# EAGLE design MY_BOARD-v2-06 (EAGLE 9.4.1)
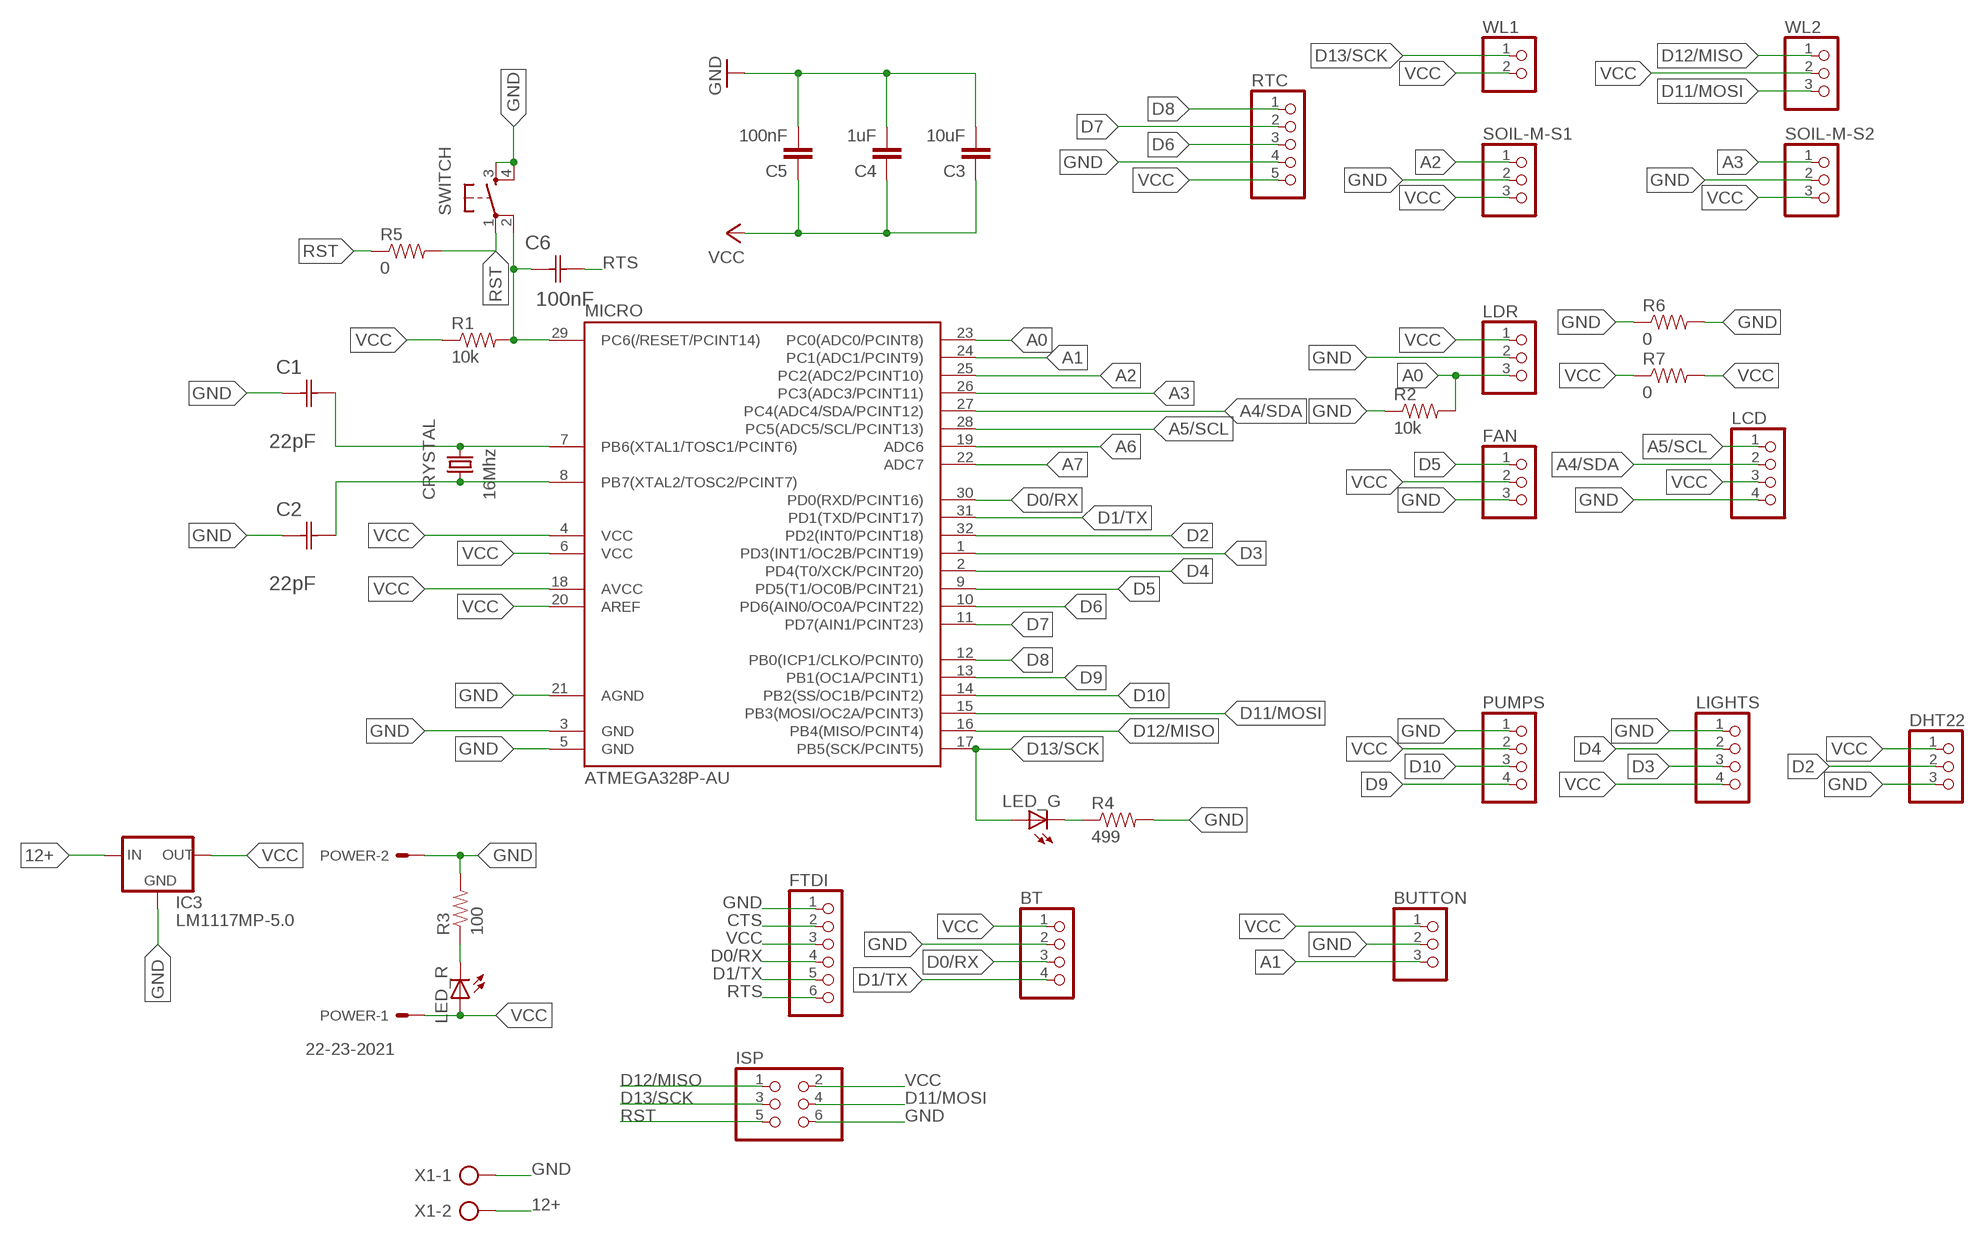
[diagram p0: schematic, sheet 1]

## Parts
BT  PINHD-1X4/90  [1X04/90]
BUTTON  PINHD-1X3/90  [1X03/90]
C1  22pF  0612ZC225MAT2A  [CAPC3216X178N]
C2  22pF  0612ZC225MAT2A  [CAPC3216X178N]
C3  10uF  CAP1206  [1206]
C4  1uF  CAP1206  [1206]
C5  100nF  CAP1206  [1206]
C6  100nF  0612ZC225MAT2A  [CAPC3216X178N]
CRYSTAL  16Mhz  CSM-7X-DU  [CSM-7X-DU]
DHT22  PINHD-1X3/90  [1X03/90]
FAN  PINHD-1X3/90  [1X03/90]
FTDI  PINHD-1X6  [1X06]
IC3  LM1117MP-5.0  [SOT223]
ISP  PINHD-2X3-SMD  [2X03SMD]
LCD  PINHD-1X4/90  [1X04/90]
LDR  PINHD-1X3/90  [1X03/90]
LED_G  LED1206  [1206]
LED_R  LED1206  [1206]
LIGHTS  PINHD-1X4/90  [1X04/90]
MICRO  ATMEGA328P-AU  ATMEGA48/88/168-AU  [TQFP32-08]
POWER  22-23-2021  [22-23-2021]
PUMPS  PINHD-1X4/90  [1X04/90]
R1  10k  RESISTOR1206  [1206]
R2  10k  RESISTOR1206  [1206]
R3  100  RESISTOR1206  [1206]
R4  499  RESISTOR1206  [1206]
R5  0  RESISTOR1206  [1206]
R6  0  RESISTOR1206  [1206]
R7  0  RESISTOR1206  [1206]
RTC  PINHD-1X5/90  [1X05/90]
SOIL-M-S1  PINHD-1X3/90  [1X03/90]
SOIL-M-S2  PINHD-1X3/90  [1X03/90]
SWITCH  6MM_SWITCH6MM_SWITCH  [6MM_SWITCH]
WL1  PINHD-1X2/90  [1X02/90]
WL2  PINHD-1X3/90  [1X03/90]
X1  AK500/2  [AK500/2]

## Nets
12+: IC3.3(IN) X1.2
A0: LDR.3 MICRO.23(PC0(ADC0/PCINT8)) R2.2
A1: BUTTON.3 MICRO.24(PC1(ADC1/PCINT9))
A2: MICRO.25(PC2(ADC2/PCINT10)) SOIL-M-S1.1
A3: MICRO.26(PC3(ADC3/PCINT11)) SOIL-M-S2.1
A4/SDA: LCD.2 MICRO.27(PC4(ADC4/SDA/PCINT12))
A5/SCL: LCD.1 MICRO.28(PC5(ADC5/SCL/PCINT13))
A6: MICRO.19(ADC6)
A7: MICRO.22(ADC7)
CTS: FTDI.2
D0/RX: BT.3 FTDI.4 MICRO.30(PD0(RXD/PCINT16))
D1/TX: BT.4 FTDI.5 MICRO.31(PD1(TXD/PCINT17))
D2: DHT22.2 MICRO.32(PD2(INT0/PCINT18))
D3: LIGHTS.3 MICRO.1(PD3(INT1/OC2B/PCINT19))
D4: LIGHTS.2 MICRO.2(PD4(T0/XCK/PCINT20))
D5: FAN.1 MICRO.9(PD5(T1/OC0B/PCINT21))
D6: MICRO.10(PD6(AIN0/OC0A/PCINT22)) RTC.3
D7: MICRO.11(PD7(AIN1/PCINT23)) RTC.2
D8: MICRO.12(PB0(ICP1/CLKO/PCINT0)) RTC.1
D9: MICRO.13(PB1(OC1A/PCINT1)) PUMPS.4
D10: MICRO.14(PB2(SS/OC1B/PCINT2)) PUMPS.3
D11/MOSI: ISP.4 MICRO.15(PB3(MOSI/OC2A/PCINT3)) WL2.3
D12/MISO: ISP.1 MICRO.16(PB4(MISO/PCINT4)) WL2.1
D13/SCK: ISP.3 LED_G.1(A) MICRO.17(PB5(SCK/PCINT5)) WL1.1
GND: BT.2 BUTTON.2 C1.1(C1) C2.1(C1) C3.2 C4.2 C5.2 DHT22.3 FAN.3 FTDI.1 IC3.1(GND) ISP.6 LCD.4 LDR.2 LIGHTS.1 MICRO.3(GND) MICRO.5(GND) MICRO.21(AGND) POWER.2 PUMPS.1 R2.1 R3.2 R4.2 R6.1 R6.2 RTC.4 SOIL-M-S1.2 SOIL-M-S2.2 SWITCH.3(S) SWITCH.4(S1) X1.1
LED: LED_R.2(C) R3.1
LED1: LED_G.2(C) R4.1
RST: C6.1(C1) ISP.5 MICRO.29(PC6(/RESET/PCINT14)) R1.2 R5.1 R5.2 SWITCH.1(P) SWITCH.2(P1)
RTS: C6.2(C2) FTDI.6
VCC: BT.1 BUTTON.1 C3.1 C4.1 C5.1 DHT22.1 FAN.2 FTDI.3 IC3.2(OUT) IC3.4(OUT) ISP.2 LCD.3 LDR.1 LED_R.1(A) LIGHTS.4 MICRO.4(VCC) MICRO.6(VCC) MICRO.18(AVCC) MICRO.20(AREF) POWER.1 PUMPS.2 R1.1 R7.1 R7.2 RTC.5 SOIL-M-S1.3 SOIL-M-S2.3 WL1.2 WL2.2
XTAL1: C1.2(C2) CRYSTAL.2 MICRO.7(PB6(XTAL1/TOSC1/PCINT6))
XTAL2: C2.2(C2) CRYSTAL.1 MICRO.8(PB7(XTAL2/TOSC2/PCINT7))

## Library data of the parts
BT LCD LIGHTS PUMPS = pinhead:PINHD-1X4: PIN HEADER
BUTTON DHT22 FAN LDR SOIL-M-S1 SOIL-M-S2 WL2 = pinhead:PINHD-1X3: PIN HEADER
C1 C2 C6 = AVX_By_element14_Batch_1:0612ZC225MAT2A: Capacitor 1206; MPN: 0612ZC225MAT2A; OC_FARNELL: -; OC_NEWARK: 12N3209; SUPPLIER: AVX; TOLERANCE: ±20%; VALUE: 2.2µF; VOLTAGERATING: 10V
C3-C5 = 01_SparkFun:CAP: Capacitor
CRYSTAL = 01_FAB_Hello:CSM-7X-DU: SMD CRYSTAL; OC_FARNELL: unknown; OC_NEWARK: unknown
FTDI = pinhead:PINHD-1X6: PIN HEADER
IC3 = lm1117:LM1117?-*: 800mA Low-Dropout Linear Regulator Source: http://ww1.microchip.com/downloads/en/DeviceDoc/39760d.pdf; MF: Texas Instruments; MPN: LM1117MP-5.0; OC_FARNELL: 9778209; OC_NEWARK: 28X3417; SPICEPREFIX: J
ISP = fab:PINHD-2X3-SMD: PIN HEADER
LED_G LED_R = 01_FAB_Hello:LED
MICRO = atmega8:ATMEGA48/88/168
POWER = con-molex:22-23-2021: .100" (2.54mm) Center Header - 2 Pin; MF: MOLEX; MPN: 22-23-2021; OC_FARNELL: 1462926; OC_NEWARK: 25C3832
R1-R7 = 01_SparkFun:RESISTOR: Resistor
RTC = pinhead:PINHD-1X5: PIN HEADER
SWITCH = 01_FAB_Hello:6MM_SWITCH: OMRON SWITCH
WL1 = pinhead:PINHD-1X2: PIN HEADER
X1 = con-ptr500:AK500/2: CONNECTOR; OC_FARNELL: unknown; OC_NEWARK: unknown

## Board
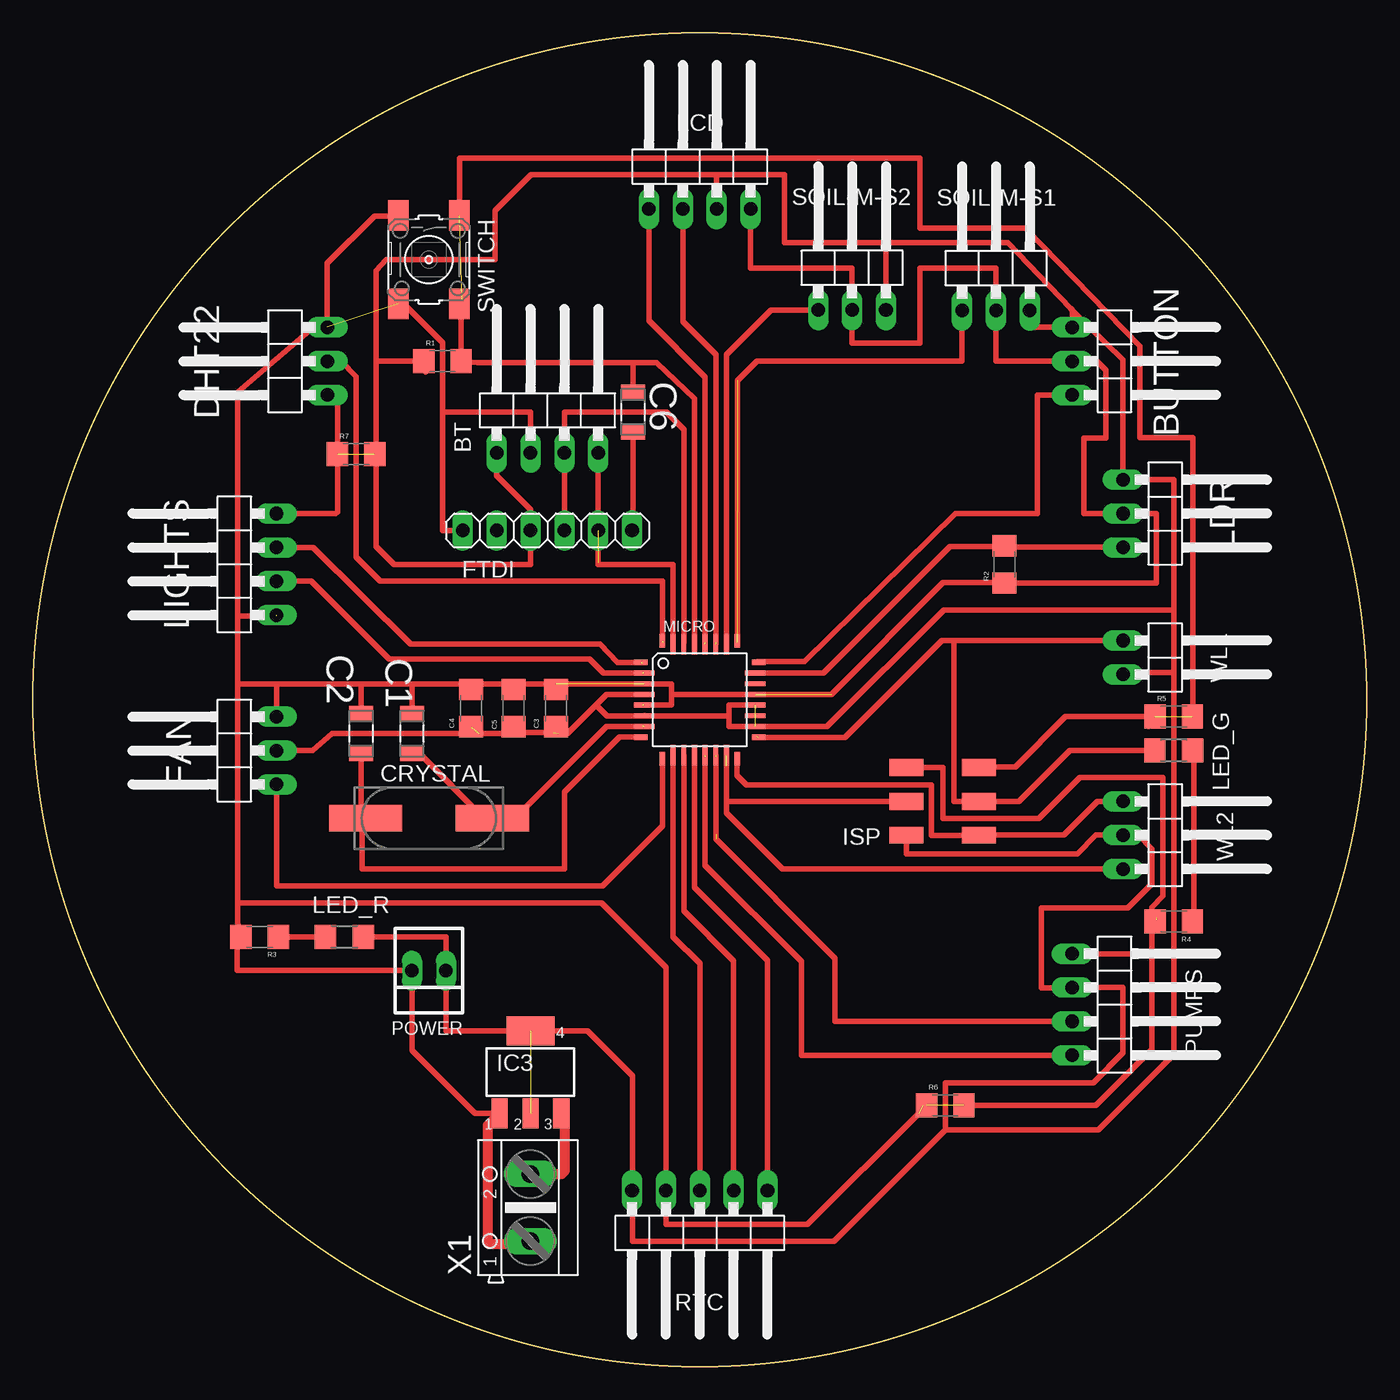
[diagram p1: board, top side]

Size 100 x 100 mm. Coordinates in mm from the lower left corner, seen from the top.
Outline: circle at 50,50 radius 50
Copper layers (1*16): Top 0.035mm / dielectric 1.5mm / Bottom 0.035mm
Design rules "default *": minimum track width 16mil, minimum drill 0.35mm, track to track 16mil, track to pad 16mil, pad to pad 16mil, via to via 16mil, smd to smd 6mil, copper to edge 40mil, drill to drill 6mil, minimum pad ring 10mil, minimum via ring 8mil, stop-mask expansion 4mil, vias tented up to drill 0mil, thermal gap 10mil

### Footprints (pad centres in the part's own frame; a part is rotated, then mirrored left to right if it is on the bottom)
1X04/90 = drill 1.016 long: 1 -3.81,-3.81; 2 -1.27,-3.81; 3 1.27,-3.81; 4 3.81,-3.81
1X03/90 = drill 1.016 long: 1 -2.54,-3.81; 2 0,-3.81; 3 2.54,-3.81
CAPC3216X178N = smd 1.118 x 1.803: 1 -1.499,0; 2 1.499,0
1206 = smd 1.6 x 1.8: 1 -1.4,0; 2 1.4,0
CSM-7X-DU = smd 5.5 x 2: 1 -4.75,0; 2 4.75,0
1X06 = drill 1.016 long: 1 -6.35,0; 2 -3.81,0; 3 -1.27,0; 4 1.27,0; 5 3.81,0; 6 6.35,0
SOT223 = smd 1.219 x 2.235: 1 -2.311,-3.099; 2 0,-3.099; 3 2.311,-3.099 | smd 3.6 x 2.2: 4 0,3.099
2X03SMD = smd 2.54 x 1.27: 1 -2.54,2.54; 2 2.92,2.54; 3 -2.54,0; 4 2.92,0; 5 -2.54,-2.54; 6 2.92,-2.54
1206' = smd 1.6 x 1.803: 1 -1.422,0; 2 1.422,0
TQFP32-08 = smd 1.016 x 0.406: 1 -4.42,2.8; 8 -4.42,-2.8; 17 4.42,-2.8; 24 4.42,2.8 | smd 1.524 x 0.356: 2 -4.166,2; 3 -4.166,1.2; 4 -4.166,0.4; 5 -4.166,-0.4; 6 -4.166,-1.2; 7 -4.166,-2; 18 4.166,-2; 19 4.166,-1.2; 20 4.166,-0.4; 21 4.166,0.4; 22 4.166,1.2; 23 4.166,2 | smd 0.406 x 1.016: 9 -2.8,-4.42; 16 2.8,-4.42; 25 2.8,4.42; 32 -2.8,4.42 | smd 0.356 x 1.524: 10 -2,-4.166; 11 -1.2,-4.166; 12 -0.4,-4.166; 13 0.4,-4.166; 14 1.2,-4.166; 15 2,-4.166; 26 2,4.166; 27 1.2,4.166; 28 0.4,4.166; 29 -0.4,4.166; 30 -1.2,4.166; 31 -2,4.166
22-23-2021 = drill 1 long: 1 -1.27,0; 2 1.27,0
1X05/90 = drill 1.016 long: 1 -5.08,-3.81; 2 -2.54,-3.81; 3 0,-3.81; 4 2.54,-3.81; 5 5.08,-3.81
6MM_SWITCH = smd 2.286 x 1.524: 1 -3.302,2.286; 2 3.302,2.286; 3 -3.302,-2.286; 4 3.302,-2.286
1X02/90 = drill 1.016 long: 1 -1.27,-3.81; 2 1.27,-3.81
AK500/2 = drill 1.321 long: 1 -2.515,0; 2 2.515,0

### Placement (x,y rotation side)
BT  38.57,72.35 0 top
BUTTON  81.75,75.4 270 top
C1  28.41,47.46 270 top
C2  24.6,47.46 270 top
C3  39.2,49.37 90 top
C4  32.86,49.37 90 top
C5  36.03,49.37 90 top
C6  45,71.59 270 top
CRYSTAL  29.68,41.11 0 top
DHT22  18.25,75.4 90 top
FAN  14.44,46.19 90 top
FTDI  38.57,62.7 0 top
IC3  37.3,22.06 0 top
ISP  68.41,42.38 180 top
LCD  50,90.64 0 top
LDR  85.56,63.97 270 top
LED_G  [1206']  85.56,46.19 0 top
LED_R  [1206']  23.33,32.22 180 top
LIGHTS  14.44,60.16 90 top
MICRO  50,50 0 top
POWER  29.68,29.68 180 top
PUMPS  81.75,27.14 270 top
R1  30.7,75.4 0 top
R2  72.86,60.16 90 top
R3  16.98,32.22 180 top
R4  85.56,33.36 180 top
R5  85.56,48.73 0 top
R6  68.41,19.57 0 top
R7  24.22,68.41 0 top
RTC  50,9.36 180 top
SOIL-M-S1  72.22,83.02 0 top
SOIL-M-S2  61.43,83.05 0 top
SWITCH  29.68,83.02 270 top
WL1  85.56,53.17 270 top
WL2  85.56,39.84 270 top
X1  37.3,11.9 90 top

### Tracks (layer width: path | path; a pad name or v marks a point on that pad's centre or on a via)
12+
  Top 0.406: 39.66,14.41 39.84,14.59
  Top 0.762: IC3.3 39.84,18.73 39.84,14.59 | X1.2 39.66,14.41
A0
  Top 0.406: MICRO.23 59.27,52 68.75,61.48 72.88,61.48 R2.2 | 73.07,61.2 R2.2 | LDR.3 81.72,61.46 73.01,61.46 R2.2
A1
  Top 0.406: BUTTON.3 75.32,72.86 75.32,63.97 69.18,63.97 57.86,52.85 54.34,52.85 54.29,52.8
A2  (1 unrouted)
  Top 0.406: 52.82,54.42 52.82,73.93 54.29,75.4 69.69,75.4 SOIL-M-S1.1
A3
  Top 0.406: SOIL-M-S2.1 55.34,79.23 52,75.89 52,54.29
A4/SDA  (1 unrouted)
  Top 0.406: MICRO.27 51.2,75.91 48.73,78.38 LCD.2
A5/SCL  (1 unrouted)
  Top 0.406: MICRO.28 50.4,74.22 46.19,78.43 LCD.1
D0/RX
  Top 0.406: 48.8,54.29 48.8,70.27 47.5,71.59 39.84,71.59 39.84,68.92 BT.3 | BT.3 39.82,67.93 | FTDI.4 BT.3
D1/TX  (1 unrouted)
  Top 0.406: 48,54.29 48,60.16 42.38,60.16 FTDI.5 | BT.4 42.38,60.29
D2  (1 unrouted)
  Top 0.406: DHT22.2 23.08,75.4 24.22,74.26 24.22,60.69 26.02,58.89 47.2,58.89 MICRO.32
D3  (1 unrouted)
  Top 0.406: LIGHTS.3 21,61.43 28.32,54.19 42.51,54.19 43.82,52.8 MICRO.1
D4  (1 unrouted)
  Top 0.406: LIGHTS.2 20.84,58.89 26.68,53.05 41.72,53.05 42.77,52 MICRO.2
D5
  Top 0.406: FAN.1 18.25,36.03 42.72,36.03 47.2,40.51 47.2,45.71
D6
  Top 0.406: RTC.3 50,30.21 48,32.21 MICRO.10
D7
  Top 0.406: MICRO.11 48.8,34.15 52.54,30.41 RTC.2
D8
  Top 0.406: 49.61,45.82 MICRO.12 49.6,35.92 55.08,30.44 RTC.1
D9  (1 unrouted)
  Top 0.406: PUMPS.4 57.62,23.33 57.62,30.37 50.4,37.59 MICRO.13
D10  (2 unrouted)
  Top 0.406: MICRO.14 51.2,39.91 | PUMPS.3 60.16,25.87 60.16,30.59 51.21,39.54 51.21,39.91
D11/MOSI  (1 unrouted)
  Top 0.406: ISP.4 52,42.38 | 52,45.03 52,42.38 | 52,42.38 52,41.52 56.22,37.3 WL2.3
D12/MISO
  Top 0.406: MICRO.16 52.8,44.34 53.51,43.62 67.37,43.62 67.37,39.83 69.8,39.83 ISP.1 77.31,39.84 79.84,42.38 WL2.1
D13/SCK  (1 unrouted)
  Top 0.406: 69.08,54.45 69.08,42.38 ISP.3 73.95,42.38 77.76,46.19 LED_G.1 | 54.42,47.19 60.9,47.19 68.16,54.45 69.08,54.45 | 69.08,54.45 WL1.1
GND  (9 unrouted)
  Top 0.406: 24.6,51.2 18.38,51.2 | 18.38,51.2 15.33,51.2 | C2.1 24.6,51.2 | C1.1 28.41,51.2 | 39.2,51.2 36.66,51.2 | 36.66,51.2 33.36,51.2 | 15.33,34.76 15.33,51.2 | 30.7,71.59 30.7,62.7 FTDI.1 | 30.7,71.59 30.7,76.8 27.8,79.72 SWITCH.4 | SWITCH.3 27.95,86.3 25.61,86.3 22.06,82.75 DHT22.3 21.02,77.94 15.33,73.09 15.33,56.3 | 83.91,30.95 83.91,23.76 79.72,19.57 R6.2 | 18.25,56.3 15.33,56.3 | 15.33,34.76 42.63,34.76 47.46,29.93 RTC.4 47.46,10.63 58.1,10.63 66.41,18.94 | ISP.6 68.24,44.92 68.24,41.11 75.45,41.11 78.52,44.18 84.74,44.18 84.74,35.27 83.91,34.43 83.91,33.24 | R6.1 66.76,19.57 | 15.33,34.76 15.33,33.24 R3.2 15.27,31.91 15.27,29.68 POWER.2 28.41,23.71 33.16,18.96 IC3.1 | PUMPS.1 83.91,30.95 | 84.29,33.49 R4.2 | FAN.3 18.25,51.07 18.38,51.2 | 15.33,56.3 15.33,51.2 | 83.91,30.95 83.91,33.24 | 83.91,33.24 84.29,33.62 | C4.2 33.36,50.64 33.36,51.2 | 33.36,51.2 33.36,51.23 | C5.2 36.66,51.2 | C3.2 39.2,51.2 | 47.88,50.4 59.87,50.4 68.26,58.78 72.84,58.78 R2.1 72.87,58.74 84.27,58.74 84.27,63.97 LDR.2 78.8,63.97 78.8,69.63 80.48,69.63 80.48,74.75 79.78,75.4 BUTTON.2 72.22,75.4 SOIL-M-S1.2 72.22,82.38 66.51,82.38 66.51,76.77 61.43,76.77 SOIL-M-S2.2 61.43,82.38 53.81,82.38 LCD.4 | 45.71,49.6 47.84,49.6 47.88,49.64 47.88,50.4 | 39.2,51.2 47.88,51.2 47.88,50.4 | 30.7,71.59 37.3,71.59 BT.2 37.28,68.56 | 24.6,51.2 28.41,51.2 | 28.41,51.2 33.36,51.2 | 37.1,9.18 X1.1
  Top 0.762: IC3.1 34.1,18.07 34.1,9.18 37.1,9.18
LED
  Top 0.406: R3.1 LED_R.2
LED1
  Top 0.406: 86.98,45.43 LED_G.2 86.83,46.17 87.09,45.91 87.09,33.49 R4.1 86.98,33.39
RST  (2 unrouted)
  Top 0.406: 32.15,79.94 SWITCH.2 32.1,79.59 R1.2 33.33,75.3 45.02,75.3 | 45.02,75.3 46.75,75.3 49.6,72.6 49.6,54.29 | ISP.5 70.12,44.97 73.67,44.97 77.43,48.73 R5.1 83.66,47.98 | SWITCH.1 31.97,90.64 66.51,90.64 66.51,85.37 74.45,85.37 83.02,76.54 83.02,69.69 87.01,69.69 87.01,48.74 R5.2 | C6.1 45,75.27 45.02,75.3
RTS
  Top 0.406: 44.95,70.04 C6.2 45,62.78 FTDI.6
VCC  (5 unrouted)
  Top 0.406: 54.18,49.59 MICRO.20 52.21,49.6 52.21,48.8 | 45.85,48.81 MICRO.6 | 85.56,56.73 68.33,56.73 59.53,48 52.21,48 52.21,48.8 | 29.43,74.59 R1.1 25.72,75.4 | MICRO.4 45.83,50.38 42.99,50.38 42.23,49.62 | MICRO.6 52.21,48.8 | 44.95,15.73 RTC.5 44.95,15.69 | 85.56,52.03 85.56,23.38 79.9,17.72 68.41,17.72 | 85.56,56.73 85.56,52.03 | 68.41,17.72 68.41,21.27 79.52,21.27 81.75,23.51 81.75,28.41 PUMPS.2 77.95,28.39 75.63,28.39 75.63,34.38 82.12,34.38 83.92,36.19 83.92,38.81 82.89,39.84 WL2.2 79.72,39.84 78.32,38.44 65.49,38.44 65.5,38.44 ISP.2 | 44.95,15.69 44.95,9.36 60.06,9.36 68.41,17.72 | BUTTON.1 79.22,77.94 81.75,75.52 LDR.1 85.56,66.51 85.56,56.73 | 79.18,77.94 77.81,79.37 | 77.81,79.37 73.11,84.29 63.97,84.29 | FTDI.3 37.27,61.4 | POWER.1 30.95,25.16 IC3.4 | BUTTON.1 74.77,77.94 SOIL-M-S1.3 | WL1.2 81.88,52.03 85.56,52.03 | 25.72,75.4 25.72,82.2 26.46,83.02 34.63,83.02 34.63,86.7 37.33,89.4 51.3,89.4 | LIGHTS.4 22.7,63.97 22.82,64.1 R7.1 | 22.7,72.86 22.82,72.86 R7.1 | 22.7,72.86 DHT22.1 | FAN.2 20.95,46.19 22.42,47.46 33.44,47.46 | 33.44,47.46 33.52,47.49 | POWER.1 30.95,32.22 LED_R.1 | 44.95,15.69 44.95,21.78 41.57,25.16 IC3.4 | 42.23,49.62 40.09,47.48 39.69,47.48 C3.1 39.37,47.8 39.37,47.48 | 42.23,49.62 43.05,48.8 MICRO.6 | IC3.4 36.59,25.87 | 30.95,25.87 POWER.1 | 22.82,72.74 22.7,72.86 | BUTTON.1 77.94,79.24 77.81,79.37 | BT.1 34.76,66.81 37.3,64.27 FTDI.3 | R7.1 | 25.87,68.67 25.72,68.51 | 25.72,68.51 R7.2 | SOIL-M-S2.3 63.97,84.29 | 51.3,89.4 51.27,89.37 LCD.3 | FTDI.3 37.3,60.16 27.06,60.16 25.72,61.51 25.72,68.51 | 25.72,75.4 25.72,68.51 | 33.44,47.46 35.78,47.46 C5.1 36.21,47.53 39.03,47.53
  Top 0.406: 51.3,89.4 56.35,89.4 56.35,84.29 63.97,84.29
XTAL1  (1 unrouted)
  Top 0.406: MICRO.7 43.02,48 36.18,41.16 35.32,41.16 CRYSTAL.2 33.82,41.11 28.97,45.96 C1.2
XTAL2
  Top 0.406: C2.2 24.6,41.44 CRYSTAL.1 24.65,40.83 24.65,37.3 39.84,37.3 39.84,43.07 43.97,47.2 45.71,47.2

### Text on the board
TEXT: LCD | SM2 | SM1 | BT | PB | DHT22 | LDR | G | LIGHTS | FTDI | WL1 | G | FAN | ISP | WL2 | B2 | 5v | G | PUMP | 12v | G | RTC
